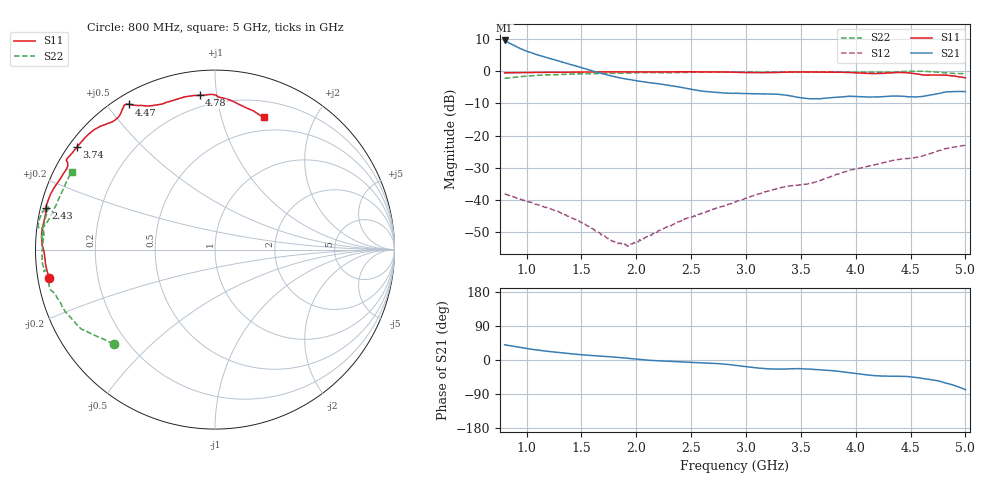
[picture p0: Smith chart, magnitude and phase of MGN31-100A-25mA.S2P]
! Port[1] = GATE
! Port[2] = DRAIN
! [Type]  S-parameter s2p file touchstone ver. 1.0
! [Object]  MGN31-100A
! [Bias]  25 mA
! [Version]  1.0
! [Date]  October, 2026
! [Source]  This file was created in JSC "ICC Milandr".
! [Disclaimer] Property of JSC "ICC Milandr". Unauthorized reproduction and/or distribution is strictly prohibited.
!  The file and the data are provided "AS IS" and with all faults and disclaim all warranties, express and implied, including
!  without limitation any implied warranties of merchantability, fitness for a particular purpose.
!  JSC "ICC Milandr" assumes no liability for:
!  1) the accuracy of the data provided;
!  2) the proper functioning of this data;
!  3) infringement of patents, copyrights or intellectual property rights resulting from the use of this data.
!  JSC "ICC Milandr" reserves the right to make changes to the products and the data without prior notice.
!  Please, be aware that your receipt and use of the file provided shall serve as acceptance of these terms and conditions.
!  If you do not accept these terms, you should return or destroy this file and any other accompanying information immediately.
# GHZ S MA R 50
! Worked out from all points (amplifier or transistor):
!   421 points, 800 MHz to 5 GHz, reference 50 ohm
!   highest |S21| = 9.5 dB at 800 MHz (marker M1)
!   |S21| within 3 dB of that: start of sweep to 978 MHz
!   unconditionally stable (mu >= 1): 1.589 GHz to 2.269 GHz
!   at 1.5 GHz: K = 0.75, MSG = 24.0 dB, |S12| = -46.9 dB
!   at 2.9 GHz: K = 0.51, MSG = 16.8 dB, |S12| = -40.6 dB
!   at 5 GHz: K = 0.72, MSG = 8.3 dB, |S12| = -23.0 dB
!   S11 on the Smith chart (normalised r, x): 800 MHz: 0.03, -0.09; 2.43 GHz: 0.01, +0.12; 3.74 GHz: 0.02, +0.33; 4.47 GHz: 0.04, +0.57; 4.78 GHz: 0.13, +0.90; 5 GHz: 0.36, +1.38
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0.8  0.9366 -170.2  2.97 40.1  0.01249 -41.0  0.7698 -137.2
0.94  0.9451 -173.9  2.245 33.0  0.01038 -46.0  0.8154 -143.5
1  0.9479 -175.4  2.031 30.2  0.009459 -47.9  0.831 -145.5
1.07  0.9492 -177.1  1.843 27.3  0.008782 -49.7  0.8476 -147.5
1.22  0.9534 -179.5  1.552 22.0  0.007346 -51.9  0.8735 -150.7
1.5  0.9642 178.1  1.126 13.9  0.004524 -47.8  0.9042 -158.2
1.78  0.9699 174.9  0.8339 8.3  0.002307 -21.4  0.9202 -163.2
1.91  0.9681 172.3  0.748 5.0  0.002001 1.3  0.9287 -165.0
2.2  0.9658 167.6  0.6348 -2.2  0.00338 47.1  0.9422 -169.1
2.43  0.972 166.3  0.5503 -5.3  0.004814 61.0  0.9502 -173.0
2.9  0.9532 157.1  0.4529 -13.9  0.009365 68.4  0.9628 -174.9
3.2  0.9419 150.7  0.441 -23.3  0.01378 62.4  0.9606 178.9
3.39  0.961 149.2  0.4156 -23.5  0.01647 64.1  0.9573 174.6
3.6  0.9639 147.4  0.3699 -24.6  0.01831 64.3  0.9685 175.3
3.74  0.9578 143.3  0.3823 -27.0  0.02217 62.7  0.9649 176.5
3.93  0.9495 135.7  0.4054 -33.1  0.02848 57.5  0.9625 174.5
4.3  0.9343 123.6  0.406 -42.7  0.03983 44.7  0.9568 165.8
4.47  0.9396 120.6  0.3996 -43.5  0.04386 42.5  0.9866 168.2
4.65  0.8636 109.1  0.4151 -50.3  0.05059 34.3  0.9858 173.2
4.78  0.8647 95.7  0.4557 -57.2  0.05958 26.5  0.9482 170.7
4.89  0.8391 84.8  0.4799 -66.3  0.06586 18.0  0.9167 163.0
5  0.7862 69.5  0.4796 -78.2  0.07082 6.1  0.9089 151.5
